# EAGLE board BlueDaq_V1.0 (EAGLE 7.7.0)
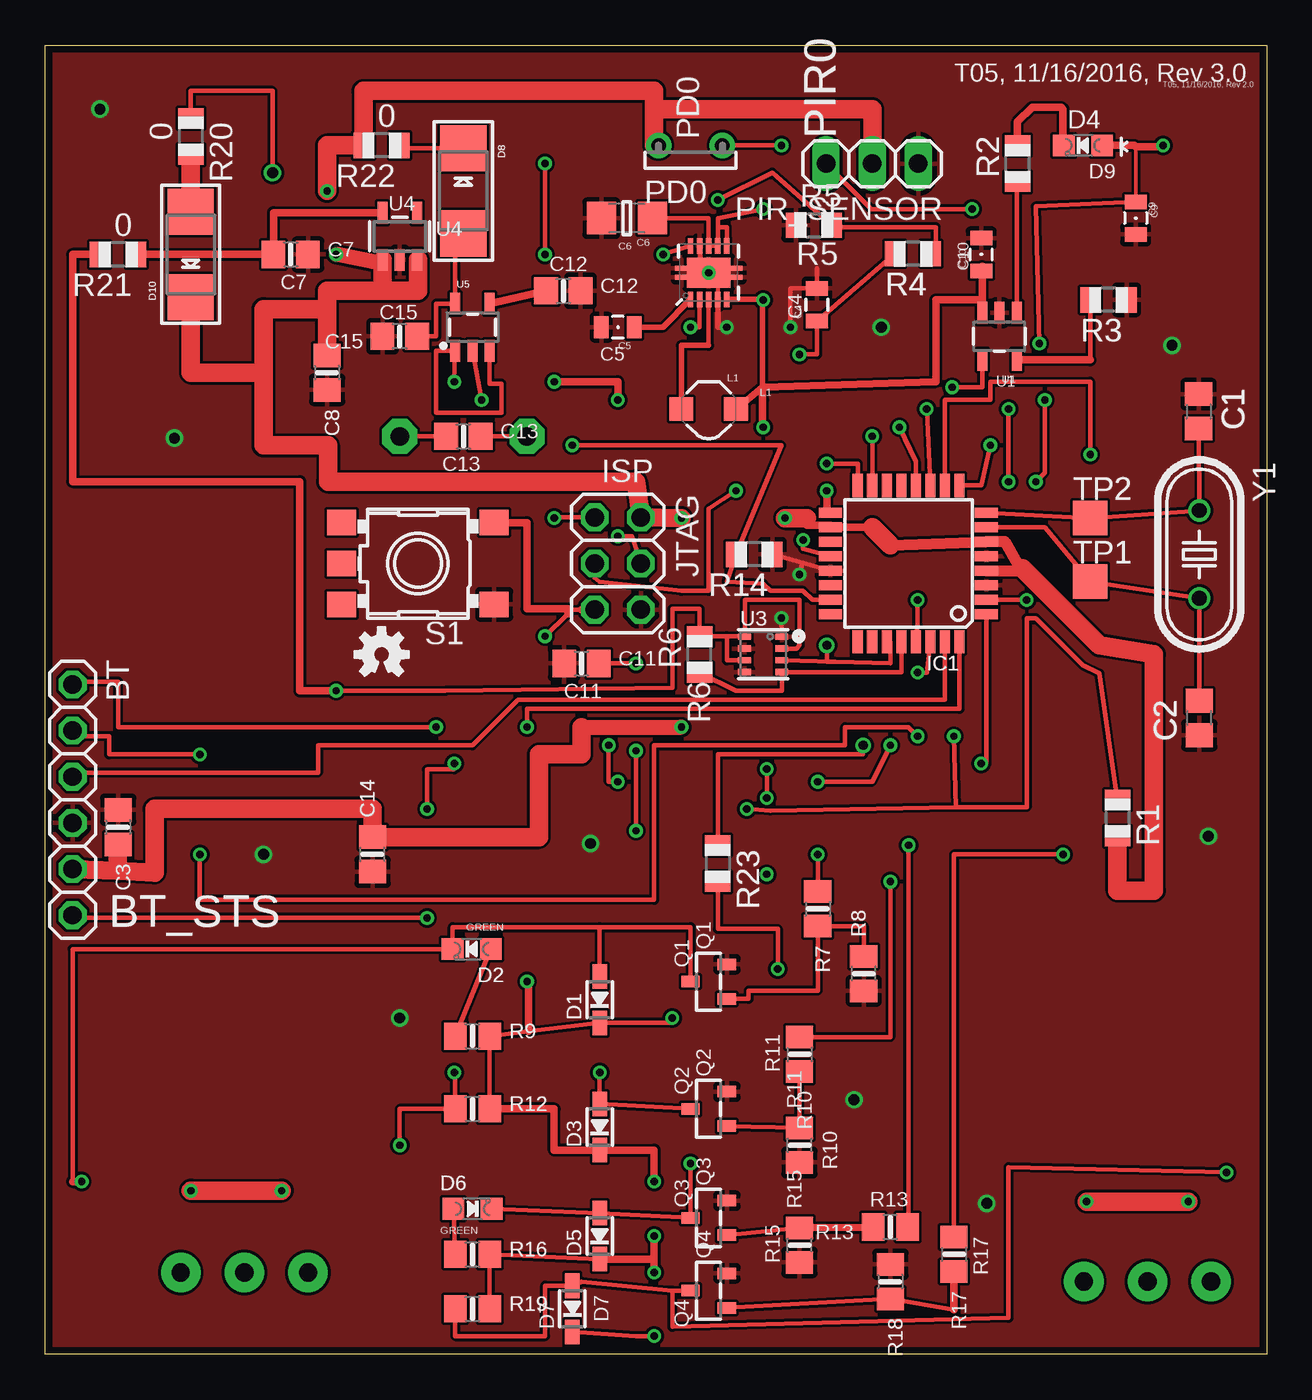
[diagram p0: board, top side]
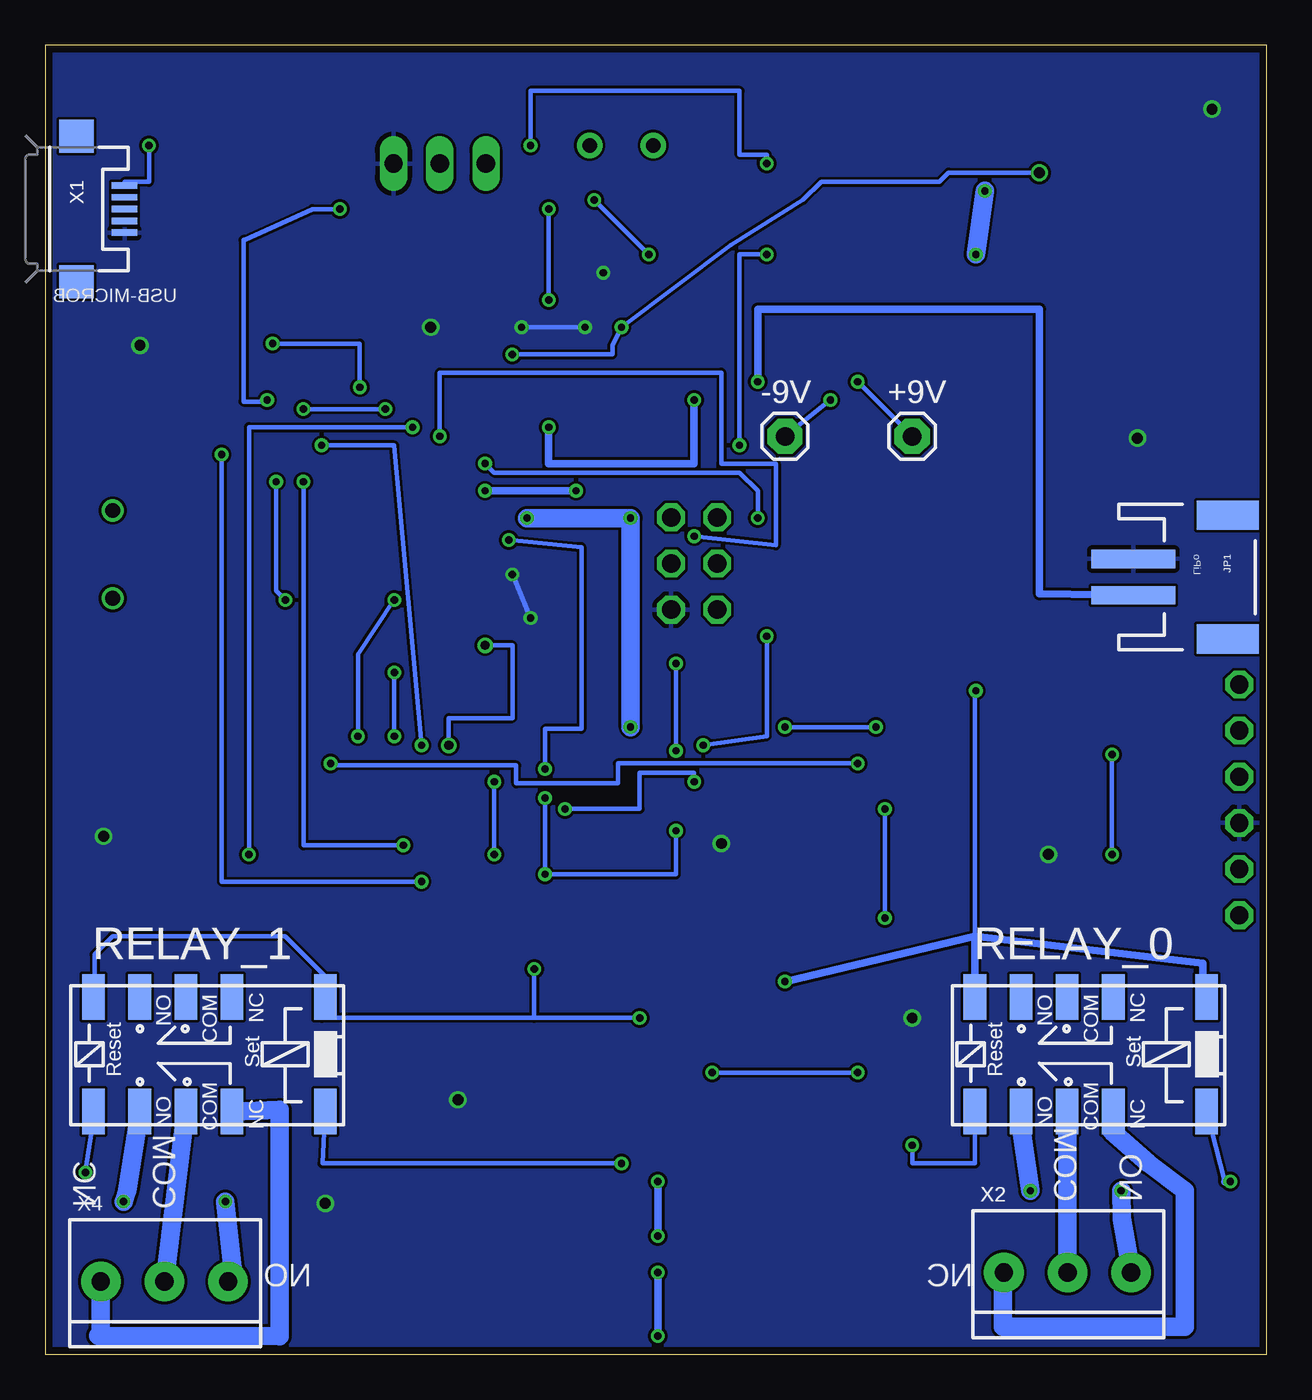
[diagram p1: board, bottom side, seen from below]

Size 67.2 x 72 mm. Coordinates in mm from the lower left corner, seen from the top.
Outline: 0,0 0,72 67.2,72 67.2,0 0,0
Copper layers (1*16): Top 0.0356mm / dielectric 1.5011mm / Bottom 0.0356mm
Design rules "OSH-Park-2-layer": minimum track width 6mil, minimum drill 13mil, track to track 6mil, track to pad 6mil, pad to pad 6mil, via to via 6mil, smd to smd 6mil, copper to edge 15mil, drill to drill 6mil, minimum pad ring 7mil, minimum via ring 7mil, stop-mask expansion 3mil, vias tented up to drill 0mil, thermal gap 10mil
Net classes: 1 HV: width 0.406 mm, drill 0.381 mm, clearance 1.016 mm

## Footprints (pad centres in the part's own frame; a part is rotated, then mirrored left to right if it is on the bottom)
1X01 = drill 1.016 pad 1.93 octagon: 1 0,0
1X06 = drill 1.016 octagon: 1 -6.35,0; 2 -3.81,0; 3 -1.27,0; 4 1.27,0; 5 3.81,0; 6 6.35,0
C0805 = smd 1.3 x 1.5: 1 -0.95,0; 2 0.95,0
0805-NO@1 = smd 1.3 x 1.5: 1 -0.95,0; 2 0.95,0
0805 = smd 0.8 x 1.2: 1 -0.9,0; 2 0.9,0
1206 = smd 1.6 x 1.8: 1 -1.4,0; 2 1.4,0
SOD-323 = smd 1.35 x 0.8: A 1.27,0; C -1.27,0
CHIPLED_0805_NOOUTLINE = smd 1.2 x 1.2: A 0,-1.05; C 0,1.05
SMADIODE = smd 2.54 x 2.54: A 2.349,0; C -2.349,0
TQFP32-08 = smd 1.27 x 0.559: 1 -4.293,2.8; 2 -4.293,2; 3 -4.293,1.2; 4 -4.293,0.4; 5 -4.293,-0.4; 6 -4.293,-1.2; 7 -4.293,-2; 8 -4.293,-2.8; 17 4.293,-2.8; 18 4.293,-2; 19 4.293,-1.2; 20 4.293,-0.4; 21 4.293,0.4; 22 4.293,1.2; 23 4.293,2; 24 4.293,2.8 | smd 0.559 x 1.27: 9 -2.8,-4.293; 10 -2,-4.293; 11 -1.2,-4.293; 12 -0.4,-4.293; 13 0.4,-4.293; 14 1.2,-4.293; 15 2,-4.293; 16 2.8,-4.293; 25 2.8,4.293; 26 2,4.293; 27 1.2,4.293; 28 0.4,4.293; 29 -0.4,4.293; 30 -1.2,4.293; 31 -2,4.293; 32 -2.8,4.293
JST-2-SMD = smd 1 x 4.6: 1 -1,-3.7; 2 1,-3.7 | smd 1.6 x 3.4: NC1 -3.4,1.5; NC2 3.4,1.5
2X03 = drill 1.016 octagon: 1 -2.54,-1.27; 2 -2.54,1.27; 3 0,-1.27; 4 0,1.27; 5 2.54,-1.27; 6 2.54,1.27
CDRH2D09 = smd 1.3 x 1.3: P$1 -1.5,0; P$2 1.5,0
M9960 = drill 0.8 pad 1.4: 1 -1.75,0; 2 1.75,0
1X03 = drill 1.016 long: 1 -2.54,0; 2 0,0; 3 2.54,0
SOT23-R = smd 0.635 x 1.016: 1 -0.95,-1; 2 0.95,-1; 3 0,1
R0805 = smd 1.1 x 1.4: 1 -1,0; 2 1,0
0805-NO = smd 1.24 x 1.5: 1 -0.95,0; 2 0.95,0
RELAY_EE2_LATCH = smd 1.25 x 2.5: 1 -6.2,-3.15; 3 -1.07,-3.15; 4 1.47,-3.15; 5 4.01,-3.15; 6 6.55,-3.15; 7 6.55,3.15; 8 4.01,3.15; 9 1.47,3.15; 10 -1.07,3.15; 12 -6.2,3.15
SKHMPXE010 = smd 1.6 x 1.4: 1 -4.2,2.25; 2 4.2,2.25; 3 -4.2,-2.25; 4 4.2,-2.25; 5 4.2,0
TP19SQ = smd 1.9 x 1.9: TP 0,0
SOT23-5 = smd 0.55 x 1.2: 1 -0.95,-1.3; 2 0,-1.3; 3 0.95,-1.3; 4 0.95,1.3; 5 -0.95,1.3
QFN-10_PAD = smd 0.297 x 0.85: 1 -1,-1.475; 2 -0.5,-1.475; 3 0,-1.475; 4 0.5,-1.475; 5 1,-1.475; 6 1,1.475; 7 0.5,1.475; 8 0,1.475; 9 -0.5,1.475; 10 -1,1.475 | smd 0.7 x 0.28: 11 -1.5,0.25; 12 -1.5,-0.25; 13 1.5,0.25; 14 1.5,-0.25 | smd 2.4 x 1.65: 15 0,0
BME280 = smd 0.7 x 0.35: 1 1.025,0.975; 2 1.025,0.325; 3 1.025,-0.325; 4 1.025,-0.975; 5 -1.025,-0.975; 6 -1.025,-0.325; 7 -1.025,0.325; 8 -1.025,0.975
USB-MICROB = smd 0.35 x 1.4: D+ 0,2.65; D- -0.65,2.65; GND 1.3,2.65; ID 0.65,2.65; VBUS -1.3,2.65 | smd 1.8 x 1.9: MT1 -4,0; MT2 4,0
TERMBLOCK_1X3-3.5MM = drill 1 pad 2.184: 1 3.55,0; 2 0.05,0; 3 -3.45,0
HC49U-V = drill 0.813: 1 -2.413,0; 2 2.413,0

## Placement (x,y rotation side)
+9V  [1X01]  19.5,50.5 0 bottom
-9V  [1X01]  26.5,50.5 0 bottom
BT  [1X06]  1.5,30.5 270 top
C1  22p  [C0805]  63.46,51.87 270 top
C2  22p  [C0805]  63.5,35 90 top
C3  0.1uF  [0805-NO@1]  4,29 270 top
C4  22uF  [0805]  42.46,57.73 90 top
C5  0.1uF  [0805]  31.5,56.5 180 top
C6  10uF  [1206]  32,62.5 180 top
C7  10uF  [0805-NO@1]  13.5,60.5 0 top
C8  10uF  [0805-NO@1]  15.5,54 270 top
C9  4.7uF  [0805]  60,62.5 270 top
C10  4.7uF  [0805]  51.5,60.5 90 top
C11  0.1uF  [0805-NO@1]  29.5,38 0 top
C12  .1uF  [0805-NO@1]  28.5,58.5 0 top
C13  10uF  [0805-NO@1]  23,50.5 0 top
C14  0.1uF  [0805-NO@1]  18,27.5 90 top
C15  10uF  [0805-NO@1]  19.5,56 180 top
D1  1N4148  [SOD-323]  30.5,19.5 90 top
D2  GREEN  [CHIPLED_0805_NOOUTLINE]  23.46,22.29 90 top
D3  1N4148  [SOD-323]  30.5,12.5 90 top
D5  1N4148  [SOD-323]  30.5,6.5 90 top
D6  GREEN  [CHIPLED_0805_NOOUTLINE]  23.5,8 270 top
D7  1N4148  [SOD-323]  29,2.5 90 top
D8  [SMADIODE]  23,64 270 top
D9  GREEN  [CHIPLED_0805_NOOUTLINE]  57.1,66.5 90 top
D10  [SMADIODE]  8,60.5 90 top
IC1  MEGA8-AI  [TQFP32-08]  47.5,43.5 180 top
JP1  LiPo  [JST-2-SMD]  3.63,42.75 270 bottom
JTAG  [2X03]  31.5,43.5 270 top
L1  4.7uH, 1.2A  [CDRH2D09]  36.5,52 0 top
PD0  M9960_11A  [M9960]  35.5,66.5 0 top
PIR_SENSOR  [1X03]  45.5,65.5 180 top
Q1  MMBT2222  [SOT23-R]  36.5,20.5 90 top
Q2  MMBT2222  [SOT23-R]  36.5,13.5 90 top
Q3  MMBT2222  [SOT23-R]  36.5,7.5 90 top
Q4  MMBT2222  [SOT23-R]  36.5,3.5 90 top
R1  10k  [R0805]  59,29.5 270 top
R2  470  [R0805]  53.5,65.5 90 top
R3  2k  [R0805]  58.5,58 180 top
R4  1.7M  [R0805]  47.74,60.54 180 top
R5  180K  [R0805]  42.29,62.11 0 top
R6  4.7k  [R0805]  36,38.5 90 top
R7  1K  [0805-NO]  42.5,24.5 270 top
R8  10K  [0805-NO]  45.03,20.94 90 top
R9  1K  [0805-NO]  23.5,17.5 0 top
R10  1K  [0805-NO]  41.5,16.5 270 top
R11  10K  [0805-NO]  41.5,11.5 90 top
R12  1K  [0805-NO]  23.5,13.5 0 top
R13  1K  [0805-NO]  46.5,7 180 top
R14  10k  [R0805]  39,44 180 top
R15  10K  [0805-NO]  41.5,6 90 top
R16  1K  [0805-NO]  23.5,5.5 0 top
R17  1K  [0805-NO]  50,5.5 270 top
R18  10K  [0805-NO]  46.5,4 270 top
R19  1K  [0805-NO]  23.5,2.5 0 top
R20  0  [R0805]  8,67 270 top
R21  0  [R0805]  4,60.5 180 top
R22  0  [R0805]  18.5,66.5 180 top
R23  4.7k  [R0805]  37,27 270 top
RELAY_0  RELAY_LATCHINGEE2NUH  [RELAY_EE2_LATCH]  9.5,16.5 180 bottom
RELAY_1  RELAY_LATCHINGEE2NUH  [RELAY_EE2_LATCH]  58,16.5 180 bottom
S1  SKHMPSE010  [SKHMPXE010]  20.5,43.5 180 top
TP1  TPTP19SQ  [TP19SQ]  57.5,42.5 0 top
TP2  TPTP19SQ  [TP19SQ]  57.5,46 0 top
U1  MCP73831  [SOT23-5]  52.5,56 180 top
U2  TPS61200  [QFN-10_PAD]  36.5,59.5 0 top
U3  BME280  [BME280]  39.5,38.5 0 top
U4  MIC5225-3.3  [SOT23-5]  19.5,61.5 0 top
U5  MIC5219 5V  [SOT23-5]  23.5,56.5 0 top
U$22  OSHW-LOGOS  [OSHW-LOGO-S]  18.5,38.5 0 top
X1  USB-MICROB  [USB-MICROB]  65.5,63 270 bottom
X2  3.5mm  [TERMBLOCK_1X3-3.5MM]  11,4.5 0 bottom
X4  3.5mm  [TERMBLOCK_1X3-3.5MM]  60.7,4 0 bottom
Y1  16 mhz  [HC49U-V]  63.5,44 270 top

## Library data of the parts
+9V -9V BT D8 D10 R1-R6 R14 R20-R23 = adafruit
C1 C2 = rcl
C3 C7 C8 C11-C15 D1-D3 D5-D7 D9 Q1-Q4 R7-R13 R15-R19 RELAY_0 RELAY_1 U3 U4 X2 X4 = microbuilder
C4 C6 = CH_passive
C5 C9 C10 JP1 L1 U1 U2 U$22 X1 = SparkFun
IC1 = atmel; MPN: ATMEGA8-16AU; OC_FARNELL: 9171371; OC_NEWARK: 73M8863
JTAG PIR_SENSOR = pinhead
PD0 = photo-elements
S1 = switch
TP1 TP2 = testpad
U5 = SparkFun-PowerIC; PROD_ID: VREG-10107
Y1 = SparkFun-FreqCtrl

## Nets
3.3V: D1.C D3.C D5.C D7.C R6.2 R9.2 R12.2 R16.2 R19.2 R21.2 R23.2 RELAY_0.1 RELAY_0.6 RELAY_1.1 RELAY_1.6 U3.2 U3.6 U3.8
BT_BRK: BT.1 IC1.32
BT_RX: BT.2 IC1.30
BT_STS: BT.6 IC1.1
BT_TX: BT.3 IC1.31
COM1 [HV]: RELAY_0.9 X2.2
COM2 [HV]: RELAY_1.9 X4.2
FB: R4.1 R5.2 U2.10
GND: BT.4 C1.1 C2.1 C3.1 C4.2 C5.2 C6.2 C7.2 C8.2 C9.2 C10.2 C11.1 C12.2 C14.1 C15.2 IC1.3 IC1.5 IC1.21 JP1.1 JTAG.6 PIR_SENSOR.1 Q1.2 Q2.2 Q3.2 Q4.2 R3.1 R5.1 R8.1 R11.1 R14.1 R15.1 R18.1 S1.1 U1.2 U2.4 U2.9 U2.11 U2.12 U2.13 U2.14 U2.15 U3.1 U3.5 U3.7 U4.2 X1.GND
N$1: IC1.23 PD0.2 R14.2
N$2: L1.P$1 U2.3
N$3: C5.1 U2.1
N$4: D9.C R2.2
N$5: C15.1 D8.A U5.5
N$6: D1.A D2.C Q1.3 RELAY_0.12
N$7: D5.A D6.C Q3.3 RELAY_1.12
N$8: Q3.1 R13.2 R15.2
N$9: D6.A R16.1
N$10 [HV]: RELAY_1.10 X4.3
N$11: R3.2 U1.5
N$12: D7.A Q4.3 R19.1 RELAY_1.7
N$13: Q4.1 R17.2 R18.2
N$14: R2.1 U1.1
N$15: +9V.1 C13.1 U5.1 U5.3
N$16: -9V.1 C13.2 U5.2
N$17: C12.1 U5.4
N$18: D8.C R22.1
N$20: D10.A R20.2
N$22: Q1.1 R7.2 R8.2
N$23: C9.1 D9.A U1.4 X1.VBUS
N$25: D3.A Q2.3 R12.1 RELAY_0.7
N$26: D2.A R9.1
N$27: Q2.1 R10.2 R11.2
N$28 [HV]: RELAY_0.10 X2.3
N$36: C11.2 IC1.20
NO1 [HV]: RELAY_0.8 X2.1
NO2 [HV]: RELAY_1.8 X4.1
OUT: C7.1 R21.1 U4.5
PIR0: IC1.2 PIR_SENSOR.3
R0_RSET: IC1.10 R10.1
R0_SET: IC1.9 R7.1
R1_RSET: IC1.12 R17.1
R1_SET: IC1.11 R13.1
RESET_PIN: IC1.29 JTAG.5 R1.1 S1.3
SCL: IC1.28 R6.1 U3.4
SDA: IC1.27 R23.1 U3.3
SPI_MISO: IC1.16 JTAG.1
SPI_MOSI: IC1.15 JTAG.4
SPI_SCK: IC1.17 JTAG.3
VBATT: C6.1 C10.1 JP1.2 L1.P$2 U1.3 U2.5 U2.6 U2.7 U2.8
VCC: BT.5 C3.2 C8.1 C14.2 D10.C IC1.4 IC1.6 IC1.18 JTAG.2 PD0.1 PIR_SENSOR.2 R1.2 R22.2 U4.1 U4.3
VOUT: C4.1 R4.2 R20.1 U2.2
XTAL1: C2.2 IC1.7 TP1.TP Y1.2
XTAL2: C1.2 IC1.8 TP2.TP Y1.1

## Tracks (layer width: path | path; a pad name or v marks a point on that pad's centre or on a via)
3.3V  (via drill 0.4)
  Top 0.254: R12.2 R9.2 26.59,17.76 D1.C 34.5,18.23 v34.5,18.5 | D5.C R16.2 R19.2 | v33.5,1 32.5,1 D7.C | v16,36.5 22,36.5 34.5,36.67 34.5,41 36,41 R6.2 37.5,39.5 | 37.5,39.5 38.45,39.5 U3.8 38.5,39.48 38.5,41.5 41.5,41.5 41.5,39 41.33,38.83 U3.2 | U3.6 37.5,38.17 37.5,39.5 | R23.2 37,23.4 40.3,23.4 v40.3,21.2
  Top 0.406: D5.C 33.5,5.23 v33.5,4.5 v33.5,6.5 | v33.5,9.5 33.5,11.23 D3.C 28,11.23 28,13.5 R12.2 | R21.2 1.5,60.5 1.5,48 14,48 14,36.5 v16,36.5 | v26.5,20.5 26.59,20.5 26.59,17.76
  Bottom 0.254: 16.05,23 16.05,36.5 v16,36.5 | v34.5,18.5 40.3,18.5 | 40.3,18.5 52,18.5 52,19.5 51.8,19.5 RELAY_1.1 51.8,20.8 54,23 63.5,23 64.5,22 64.5,19.7 RELAY_1.6 | 3.5,19.85 RELAY_0.1 | v40.3,21.2 40.3,18.5
  Bottom 0.406: RELAY_0.6 16.05,23 | 16.05,23 3.5,21.5 3.5,19.85 | v26.5,20.5 16.05,23 | v33.5,4.5 v33.5,1 | v33.5,9.5 v33.5,6.5
BT_BRK  (via drill 0.4)
  Top 0.254: IC1.32 50.3,35.5 26.5,35.5 v26.5,34.5 | v21.5,34.5 4,34.5 4,37 1.5,37 BT.1
  Bottom 0.254: v26.5,34.5 v21.5,34.5
BT_RX  (via drill 0.4)
  Top 0.254: IC1.30 48.5,37.5 v48,37.5 | v8.5,27.5 8.5,25 33.5,25 33.5,33.5 44,33.5 44,34.5 47.5,34.5 v48,34 | v8.5,33 3.5,33 3.5,34 1.5,34 BT.2
  Bottom 0.254: v48,37.5 v48,34 | v8.5,27.5 v8.5,33
BT_STS  (via drill 0.4)
  Top 0.254: IC1.1 51.79,32.5 v51.5,32.5 | v22.5,32.5 22.5,32.18 21,32.18 v21,30 | v21,24 1.5,24
  Top 0.406: 1.5,24 BT.6
  Bottom 0.254: v21,30 v21,24 | v22.5,32.5 35.7,32.5 35.7,31.4 41.3,31.4 41.3,32.4 51.5,32.4 v51.5,32.5
BT_TX
  Top 0.254: IC1.31 49.5,36 26,36 23.5,33.5 15,33.5 15,32 1.5,32 BT.3
COM1
  Bottom 1.016: X2.2 RELAY_0.9
COM2
  Bottom 1.016: X4.2 RELAY_1.9
FB  (via drill 0.4)
  Top 0.254: R4.1 49,60.5 49,62 43.29,62 R5.2 40,65 v37,63.5 | v34,60.5 U2.10
  Bottom 0.254: v37,63.5 v34,60.5
GND  (via drill 0.4, 0.6, 0.6 pad 0.25)
  Top 0.203: U2.4 37,59.5
  Top 0.254: 42.46,59.75 C4.2 41,58.63 v41,56.5 | 40,43.6 R14.1 41.65,43.54 | U3.1 v40.5,40.5 | IC1.21 41.65,43.54 | v41.5,42.9 41.65,43.54 | 37,59.5 37,59.75 U2.13 | 36.5,59.75 U2.15 36.1,59.7 | 36.1,59.7 U2.9 | 36.1,59.7 35.3,59.7 U2.11
  Top 0.305: U2.4 37,56.5 v37.5,56.5
  Bottom 0.254: v37.5,56.5 v41,56.5 | v40.5,40.5 v41.5,42.9
  other vias: 3,68.5 7.1,50.4 62,55.5 46,56.5 64,28.5 30,28.1 12,27.5 19.5,18.5 51.8,8.3 44.5,14 36.5,59.5
  pour Top: 0,0 0,72 67.2,72 67.2,0
  pour Bottom: 0,0 0,72 67.2,72 67.2,0
N$1  (via drill 0.4)
  Top 0.254: v29,50 40.5,50 R14.2 37.5,42.5 39.5,42.4 39.9,42 41.7,42 42.2,41.5 IC1.23 | v40.5,66.5 PD0.2 | v27.5,60.5 v27.5,65.5
  Bottom 0.254: v40.5,66.5 40.5,69.5 29,69.5 29,66 27.5,66 v27.5,65.5 | v29,50 29,60.5 v27.5,60.5
N$2
  Top 0.254: U2.3 36.5,55.5
  Top 0.305: 36.5,55.5 35,55.5 L1.P$1
N$3
  Top 0.305: C5.1 34,56.5 U2.1
N$4
  Top 0.406: R2.2 53.5,67.8 54.3,68.6 55.9,68.6 56,68.5 56,66.55 D9.C
N$5
  Top 0.254: D8.A 22.55,61.65 U5.5 21.5,57.8 21.5,56 C15.1
N$6  (via drill 0.4)
  Top 0.254: 30.5,23.5 22.41,23.5 D2.C 1.5,22.29 1.5,9.5 | 30.5,23.5 D1.A | 30.5,23.5 35.5,23.5 Q1.3
  Top 0.406: 1.5,9.5 v2,9.5
  Bottom 0.254: 2.3,9.5 RELAY_0.12
  Bottom 0.406: v2,9.5 2.3,9.5
N$7  (via drill 0.4)
  Top 0.254: D6.C D5.A 34.98,7.53 Q3.3 v35.5,10.5
  Bottom 0.254: RELAY_1.12 51.95,10.5 v35.5,10.5
N$8
  Top 0.254: Q3.1 R15.2
  Top 0.406: R15.2 R13.2
N$9
  Top 0.254: D6.A R16.1
N$10
  Bottom 0.406: 64.3,1.03 64.3,1.2 64.15,1.2
  Bottom 1.016: RELAY_1.10 54.3,13.45 54.3,1 64.3,1.03 | 64.15,1.2 X4.3
N$11
  Top 0.254: R3.2 57.5,54.7
  Top 0.406: 57.5,54.7 U1.5
N$12  (via drill 0.4)
  Top 0.254: R19.1 22.55,1 27.5,1 27.5,3.77 D7.A 29.5,4 34.5,3.5 | 34.5,3.5 Q4.3 | v65,10 53,10.3 53,2 34.5,1.5 34.5,3.5
  Bottom 0.254: RELAY_1.7 64.5,13.35 v65,10
N$13
  Top 0.254: Q4.1 R18.2 50,2.45
  Top 0.406: 50,2.45 R17.2
N$14
  Top 0.254: R2.1 53.45,64.5 U1.1
N$15  (via drill 0.4)
  Top 0.254: v22.5,53.5 U5.1 21.5,55.2 21.5,51.8 25.1,51.8 25.1,53.4 24.45,53.4 U5.3 | +9V.1 C13.1
  Bottom 0.254: +9V.1 v22.5,53.5
N$16  (via drill 0.4)
  Top 0.254: v24,52.5 U5.2 | C13.2 -9V.1
  Bottom 0.254: -9V.1 v24,52.5
N$17
  Top 0.406: U5.4 C12.1
N$18
  Top 0.254: D8.C 19.5,66.35 R22.1
N$20
  Top 1.016: D10.A R20.2
N$22
  Top 0.254: R8.2 45.03,23.55 R7.2 42.5,20 38.7,20 38.7,19.55 Q1.1
N$23  (via drill 0.4)
  Top 0.203: 60,66.43 C9.1
  Top 0.254: C9.1 54.5,63.15 v54.7,55.6 | v49.9,53.2 51.55,53.2 U1.4
  Top 0.406: D9.A 59.93,66.5 60,66.43 61.43,66.43 v61.5,66.5
  Bottom 0.254: v61.5,66.5 61.5,64.5 62.85,64.5 X1.VBUS | v54.7,55.6 49.9,55.6 v49.9,53.2
N$25  (via drill 0.4)
  Top 0.254: v19.5,11.5 19.5,13.5 R12.1 22.55,15.5 v22.5,15.5 | Q2.3 D3.A v30.5,15.5
  Bottom 0.254: v19.5,11.5 19.5,10.5 16.05,10.5 RELAY_0.7 | v22.5,15.5 v30.5,15.5
N$26
  Top 0.254: D2.A R9.1
N$27
  Top 0.254: Q2.1 R11.2 R10.2
N$28
  Bottom 1.016: X2.3 14.5,3.5 14.5,1.5 4.5,1.5 4.5,9 6.5,10.5 8.5,12.28 RELAY_0.10
N$36  (via drill 0.4)
  Top 0.254: IC1.20 41.7,44.3 v41.7,44.8 | v32.5,28.8 v32.5,33.2 | v32.5,38 C11.2 | v39.7,32.2 v39.7,30.6
  Bottom 0.254: v41.7,44.8 37.7,44.4 37.7,34.4 39.7,34.4 v39.7,32.2 | v32.5,28.8 32.5,26.4 v39.7,26.4 v39.7,30.6 | v32.5,33.2 v32.5,38
NO1  (via drill 0.4)
  Top 1.016: v8,9 v13,9
  Bottom 1.016: RELAY_0.8 13.5,12.34 v13,9 | X2.1 7.95,7.45 v8,9
NO2  (via drill 0.4)
  Top 1.016: v62.9,8.4 v57.3,8.4
  Bottom 0.406: 56.8,4 X4.1
  Bottom 1.016: RELAY_1.8 62.71,9 v62.9,8.4 | v57.3,8.4 56.8,4
OUT
  Top 0.406: R21.1 C7.1 12.55,62.8 U4.5
PIR0  (via drill 0.4)
  Top 0.254: IC1.2 v54,41.5 | v54.5,48 55,48.5 v55,52.5 | v51,63 45.46,63 PIR_SENSOR.3
  Bottom 0.254: v54,41.5 54.5,42 v54.5,48 | v51,63 52.5,63 56.2,61.3 56.3,61.3 56.3,52.4 55,52.4 v55,52.5
R0_RSET  (via drill 0.4)
  Top 0.254: IC1.10 49.5,52.5 52,52.5 52,53.5 57.5,53.5 v57.5,49.5 | v46.5,26 46.5,17.45 R10.1
  Bottom 0.254: v57.5,49.5 57.5,26 v46.5,26
R0_SET  (via drill 0.4)
  Top 0.254: R7.1 v42.5,27.5 | v42.5,31.5 45.5,31.5 v46.5,33.5 | v52,50 51.5,47.79 IC1.9
  Bottom 0.254: v42.5,27.5 v42.5,31.5 | v46.5,33.5 48,50 v52,50
R1_RSET  (via drill 0.4)
  Top 0.254: v47,51 47.9,49.1 IC1.12 | v56,27.5 50,27.5 R17.1
  Bottom 0.254: v56,27.5 56,51 v47,51
R1_SET  (via drill 0.4)
  Top 0.254: v48.5,52 IC1.11 | v53,48 v53,52 | R13.1 47.5,6.5 v47.5,28
  Bottom 0.254: v47.5,28 53,28 v53,48 | v48.5,52 v53,52
RESET_PIN  (via drill 0.4)
  Top 0.254: R1.1 58,37.46 57.09,37.91 54.5,40.5 54,40.5 54,30.1 50.1,30.1 | 50.1,30.1 39.9,29.9 v38.6,30 | v31.5,31.5 31,31.5 v31,33.5 | v27.5,39.5 28.75,40.75 28.96,40.96 JTAG.5 | IC1.29 48,40.11 v48,41.5 | v50,34 50.1,30.1
  Top 0.406: JTAG.5 29.49,40.96 | S1.3 26.5,45.75 26.5,41 28.75,41 28.75,40.75
  Bottom 0.254: v38.6,30 34.5,30 34.5,32 31.5,32 v31.5,31.5 | v31,33.5 27.5,34 v27.5,39.5 | v48,41.5 50,38.5 v50,34
SCL
  Top 0.254: IC1.28 47.1,37.52 U3.4 40.52,36.5 38,36.5 R6.1
SDA  (via drill 0.5)
  Top 0.254: IC1.27 46.5,39.21 46.5,38 43.49,38.09 | 43.49,38.09 U3.3 | R23.1 37,33 45,33 v45,33.5 | v43,39 43,38.09 43.49,38.09
  Bottom 0.254: v45,33.5 45,35 41.5,35 41.5,39 v43,39
SPI_MISO  (via drill 0.4)
  Top 0.254: IC1.16 44.7,49 v43,49 | v28,46 28.04,46.04 JTAG.1
  Bottom 0.254: v43,49 42.5,48.5 29,48.5 28,47.5 v28,46
SPI_MOSI  (via drill 0.4)
  Top 0.254: IC1.15 v45.5,50.5 | v31.5,45 32.27,45 JTAG.4
  Bottom 0.254: v45.5,50.5 45.5,54 30,54 30,49 27,49 27,44.5 v31.5,45
SPI_SCK  (via drill 0.4)
  Top 0.254: v38,47.5 36.5,46.5 36.5,42 35,42 30.5,42.5 30.23,42.73 JTAG.3
  Top 0.406: IC1.17 43,46.51 v43,47.5
  Bottom 0.406: v43,47.5 v38,47.5
VBATT  (via drill 0.4)
  Top 0.254: 51.55,59.85 C10.1 | U2.5 37.5,58 | C6.1 36.5,62.5 U2.8 U2.7 37,62 | 37,62 37,62.5 v39.5,63 | v39.5,58 39.5,58.02 38.5,58.02 | U2.6 37.5,62 37,62
  Top 0.305: U2.5 38.5,58.02 39.47,58.02 39.47,52.5
  Top 0.406: U1.3 51.55,58 | 51.55,58 51.55,59.85 | L1.P$2 39.47,53.2 | 39.47,53.2 49,53.5 49,58 51.55,58 | v28,53.5 31.5,53.5 v31.5,52.5 | v39.5,51 39.47,51 39.47,52.5 39.47,53.2
  Bottom 0.254: v39.5,63 v39.5,58
  Bottom 0.406: JP1.2 12.5,41.83 12.5,57.5 28,57.5 v28,53.5 | v31.5,52.5 31.5,49 39.5,49 v39.5,51
VCC  (via drill 0.4)
  Top 0.254: 33.5,66.5 PD0.1 | 53.75,43.1 53.75,43.25 | 41.9,46 41.9,45.6 | 43.21,45.6 IC1.18
  Top 0.406: 20.5,60.2 U4.3 | U4.1 18.55,60 | 45.5,45.5 IC1.18 | 43.21,45.6 41.9,45.6
  Top 0.61: 53.75,43.25 53.5,43.5 52.8,44.7 IC1.6 46.5,44.5 | IC1.4 53.75,43.1
  Top 0.813: 29.5,34.5 v35,34.5 | 18.55,60 v16,60.5
  Top 1.016: PIR_SENSOR.2 45.5,68.5 33.5,68.5 | 33.5,68.5 33.5,66.5 | 53.75,43.25 58,39 61,38.5 61,25.5 59,25.5 R1.2 | 29.5,34.5 29.5,33 27.16,33 27.16,28.45 C14.2 18,30 6,30 6,26.5 3.98,26.59 | U4.1 18.55,58.5 | 18.55,58.5 20.5,58.5 20.5,60.2 | v15.5,64 15.5,66.5 R22.2 17.5,69.5 33.5,69.5 33.5,68.5 | v35,46 JTAG.2 32.5,48 15.55,48 15.55,50 12,50 12,54 | 45.5,45.5 46.5,44.5 | 3.98,26.59 BT.5 | C8.1 15.5,57.5 | 15.5,57.5 15.5,58.5 18.55,58.5 | 12,54 12,57.5 15.5,57.5 | C3.2 3.98,28.05 3.98,26.59 | D10.C 8,54 12,54 | v40.7,46 41.9,46
  Bottom 1.016: v16,60.5 v15.5,64 | v35,34.5 v35,46 v40.7,46
VOUT  (via drill 0.4, 0.6)
  Top 0.254: R4.2 C4.1 42.46,55 v41.5,55 | U2.2 36,56.5 v35.5,56.5 | v12.5,65 12.5,69.5 8,69.5 R20.1
  Bottom 0.254: v41.5,55 36,55 36,55.5 v35.5,56.5 29.5,61 25.5,63.5 24.5,64.5 18,64.5 17.5,65 v12.5,65
XTAL1
  Top 0.254: C2.2 Y1.2 TP1.TP 55,45.5 IC1.7
XTAL2
  Top 0.254: C1.2 Y1.1 TP2.TP IC1.8

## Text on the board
tNames: T05, 11/16/2016, Rev 2.0 | PIR0 | BT_STS
_tsilk: T05, 11/16/2016, Rev 3.0 | 0 | 0 | D4 | D8 | PD0 | PIR0 | R2 | 0 | U4 | C9 | C6 | C12 | R5 | R4 | C10 | C7 | U5 | D10 | C15 | C4 | R3 | C5 | U1 | L1 | C1 | C8 | C13 | ISP | TP2 | TPTP19SQ | R14 | TP1 | TPTP19SQ | U3 | BT | IC1 | C11 | R6 | C2 | C14 | R1 | R23 | C3 | BT_STS | GREEN | R8 | R7 | D2 | Q1 | D1 | R9 | R11 | Q2 | R12 | R10 | D3 | D6 | R13 | Q3 | GREEN | R17 | R16 | D5 | R15 | R19 | D7 | R18 | Q4
_bsilk: X1 | USB-MICROB | +9V | -9V | JP1 | LiPo | RELAY_0 | RELAY_1 | NC | COM | NO | NC | COM | NO | Set | Reset | Set | Reset | COM | COM | NC | NO | NC | NO | NO | COM | X2 | COM | NC | NC | NO

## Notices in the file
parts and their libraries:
SparkFun-PowerIC: Licensing: Creative Commons ShareAlike 4.0 International - https://creativecommons.org/licenses/by-sa/4.0
